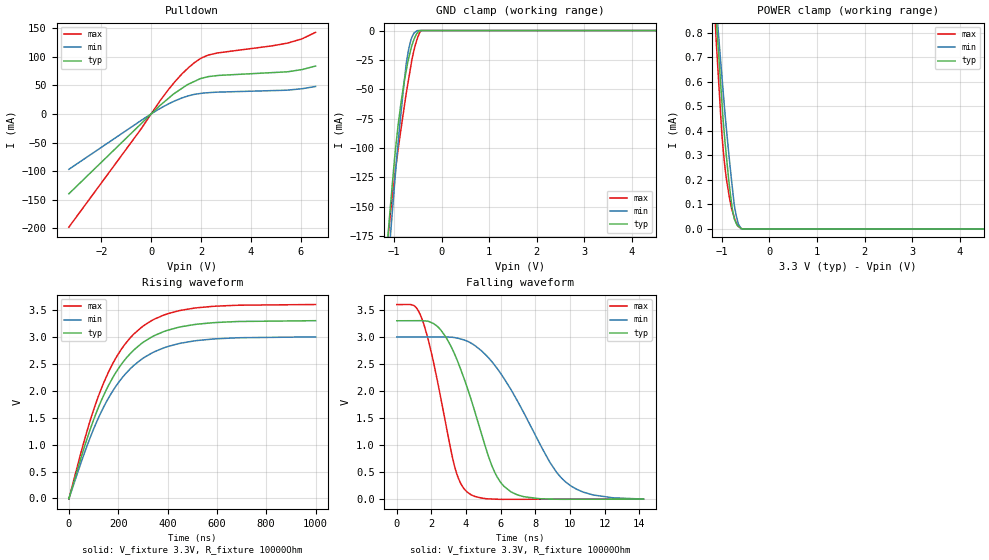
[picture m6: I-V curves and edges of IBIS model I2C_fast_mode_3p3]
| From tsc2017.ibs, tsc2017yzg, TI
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|   i2c_fast_mode_3p3 Model
[Model]   I2C_fast_mode_3p3
Model_type   I/O_open_drain
Polarity   Non-Inverting
Enable   Active-Low
Vinl = 0.99
Vinh = 2.31
Vmeas = 1.65
Vref = 3.3
Cref = 400pF
Rref = 10000
|   typ   min   max
|   (nom PVT)   (Fast PVT)   (slow PVT)
|Average
C_comp   1.438e-11   1.385e-11   1.490e-11
|ON state : BUFFER OUTPUT TURNED LOW
|C_comp   3.236e-11   3.033e-11   3.475e-11
|OFF state: BUFFER in HIGH IMPEDANCE
|C_comp   1.438e-11   1.385e-11   1.490e-11
|C_comp from frequency method(F=3.4MHz)
| Where nom  PVT is Nominal Process, 3.3V, 25C
|   Fast PVT is Strong Process,  3.6V, -40C
|   Slow PVT is Weak Process,   3V, 85C
[Model Spec]
Vinl   0.99   0.9   1.08
Vinh   2.31   2.1   2.52
[Voltage Range]   3.3   3   3.6
|Ambient Temperature   25   85   -40
|Junction Temperature
[Temperature Range]   25   85   -40
[Pullup Reference]   3.3   3   3.6
[Pulldown Reference]   0   0   0
[Power Clamp Reference]   3.3   3   3.6
[GND Clamp Reference]   0   0   0
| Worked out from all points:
|   slope of the pulldown table from 0 to 0.495 V, typ, clamps not added: 24.9 ohm
|   GND clamp passes 1 mA (typ) near -0.49 V on its own axis
|   POWER clamp passes 1 mA (typ) near -1.17 V on its own axis
|   falling waveform, V_fixture 3.3V, R_fixture 10000Ohm: 20-80 % time 2.04ns typ, 3.17ns min, 1.38ns max; typ from 3.3 V to 0.007 V
|   rising waveform, V_fixture 3.3V, R_fixture 10000Ohm: 20-80 % time 196ns typ, 203ns min, 189ns max; typ from 0.008 V to 3.3 V
[Pulldown]
|   Voltage   I(typ)   I(min)   I(max)
-3.3V     -139.5mA   -96.81mA   -197.8mA
-384mV    -16.41mA   -10.95mA   -25.15mA
368.4mV   15.2mA     9.755mA    23.5mA
663.6mV   26.06mA    16.67mA    40.79mA
1.229V    44.44mA    27.71mA    69.46mA
1.74V     56.88mA    34.22mA    89.53mA
2.024V    62.18mA    36.03mA    97.81mA
2.291V    65.14mA    37.06mA    102.9mA
2.676V    67.11mA    38.07mA    106.6mA
5.477V    73.65mA    41.56mA    123.7mA
6.064V    77.56mA    44.05mA    131.3mA
6.6V      83.68mA    47.97mA    142.6mA
[GND Clamp]
|   Voltage   I(typ)   I(min)   I(max)
-3.3V     -1.445A    -1.41A     -1.544A
-1.151V   -187.2mA   -214.2mA   -187mA
-1.096V   -159.7mA   -185.5mA   -164.7mA
-1.072V   -148.3mA   -173.3mA   -155mA
-973.5mV  -103.1mA   -124.2mA   -120.3mA
-914.1mV  -81.15mA   -96.36mA   -101.8mA
-851.4mV  -61.21mA   -69.81mA   -83.74mA
-738mV    -33.27mA   -26.88mA   -52.42mA
-627mV    -13.21mA   -5.979mA   -25.77mA
-502.8mV  -1.724mA   0A         -5.94mA
-432mV    0A         0A         0A
6.6V      0A         0A         0A
[POWER Clamp]
|   Voltage   I(typ)   I(min)   I(max)
-3.3V     7.227mA    6.118mA    8.75mA
-1.137V   912.4uA    952.9uA    834.7uA
-1.115V   847.5uA    899uA      753.3uA
-1.018V   568.8uA    665.7uA    440.8uA
-999.6mV  517.2uA    623uA      386.7uA
-973.5mV  443.8uA    561.6uA    325.7uA
-906mV    298.3uA    410.6uA    205.8uA
-778.8mV  78.64uA    166uA      72.09uA
-738mV    41.46uA    94.85uA    45.43uA
-702mV    24.37uA    56.74uA    27.51uA
-594mV    1.669uA    0A         1.83uA
6.6V      0A         0A         0A
[Ramp]
R_load = 10000
|   typ   min   max
dV/dt_r   1.9747/1.95878e-07   1.79268/2.02504e-07   2.15617/1.88934e-07
dV/dt_f   1.97542/2.04195e-09   1.79354/3.15678e-09   2.15675/1.38061e-09
[Falling Waveform]
V_fixture = 3.3V
V_fixture_min = 3V
V_fixture_max = 3.6V
R_fixture = 10000Ohm
|   Time   V(typ)   V(min)   V(max)
0s        3.3V       3V         3.6V
975ps     3.301V     3V         3.584V
1.5ns     3.3V       3.001V     3.294V
2.45ns    3.163V     3.002V     2.023V
3.35ns    2.677V     2.989V     597.9mV
4.075ns   2.059V     2.924V     134.2mV
5.5ns     616.3mV    2.542V     8.475mV
6.575ns   144.8mV    2.04V      2.79mV
9.75ns    2.709mV    323.6mV    5.356mV
14.25ns   7.309mV    6.997mV    5.494mV
[Rising Waveform]
V_fixture = 3.3V
V_fixture_min = 3V
V_fixture_max = 3.6V
R_fixture = 10000Ohm
|   Time   V(typ)   V(min)   V(max)
0s        7.62mV     10.74mV    5.411mV
81.63ns   1.218V     1.074V     1.375V
112.9ns   1.612V     1.424V     1.813V
143.1ns   1.933V     1.717V     2.166V
177.6ns   2.239V     1.992V     2.5V
213.4ns   2.493V     2.225V     2.773V
293.6ns   2.872V     2.58V      3.173V
384.4ns   3.096V     2.794V     3.402V
505.3ns   3.225V     2.922V     3.53V
1us       3.299V     2.999V     3.599V
